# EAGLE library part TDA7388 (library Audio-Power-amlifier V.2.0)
The TDA7386 is an AB class audio power amplifier, packaged in Flexiwatt 25 and designed for high end car radio applications. Based on a fully complementary PNP/NPN configuration, the TDA7386 allows a rail to rail output voltage swing with no need of bootstrap capacitors. The extremely reduced boundary components count allows very compact sets.
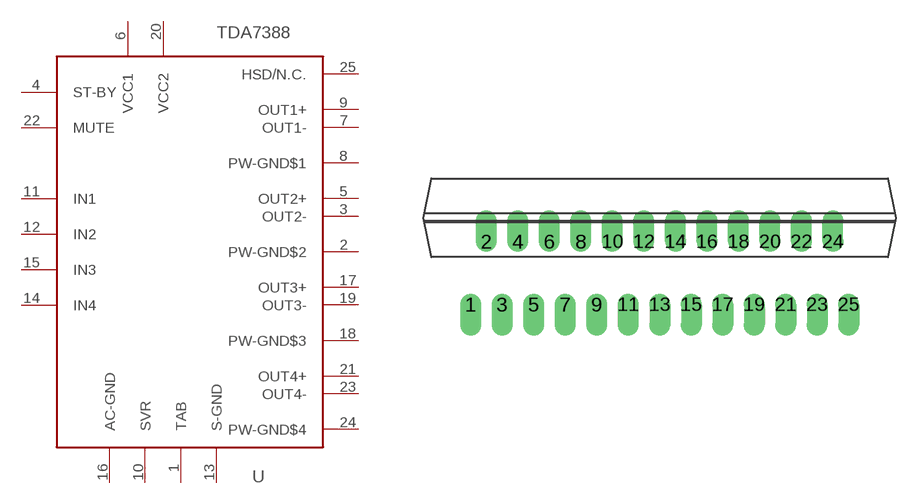
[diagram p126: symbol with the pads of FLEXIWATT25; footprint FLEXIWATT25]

Designator prefix -

## TDA7388  [FLEXIWATT25]
1  TAB
2  PW-GND$2
3  OUT2-
4  ST-BY
5  OUT2+
6  VCC1
7  OUT1-
8  PW-GND$1
9  OUT1+
10  SVR
11  IN1
12  IN2
13  S-GND
14  IN4
15  IN3
16  AC-GND
17  OUT3+
18  PW-GND$3
19  OUT3-
20  VCC2
21  OUT4+
22  MUTE
23  OUT4-
24  PW-GND$4
25  HSD/N.C.

## Footprint FLEXIWATT25 (pad centres in mm)
Flexiwatt25 (vertical)
drill 0.813 offset: 1 -12,0; 2 -11,4; 3 -10,0; 4 -9,4; 5 -8,0; 6 -7,4; 7 -6,0; 8 -5,4; 9 -4,0; 10 -3,4; 11 -2,0; 12 -1,4; 13 0,0; 14 1,4; 15 2,0; 16 3,4; 17 4,0; 18 5,4; 19 6,0; 20 7,4; 21 8,0; 22 9,4; 23 10,0; 24 11,4; 25 12,0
